(* Logix 5000 AddOnInstructionDefinition export DCO_WriteDriveParameter; software revision 20.01 *)

ADD_ON_INSTRUCTION DCO_WriteDriveParameter   (* revision 1.0 *)
// Write values to parameters in drive with data type INT and UINT
VAR_INPUT
   Instance_Number_Write : INT := 10518; {visible}
   Attribute_Number_Write : INT; {visible}
   Parameter_Value_Write : INT := 660; {visible}
   REQ_LEN : INT; {visible}
   Value_Out : INT; {visible}
END_VAR
VAR_IN_OUT
   MSG_Out : MESSAGE; {required}
END_VAR

ROUTINE Logic   (* ladder *)
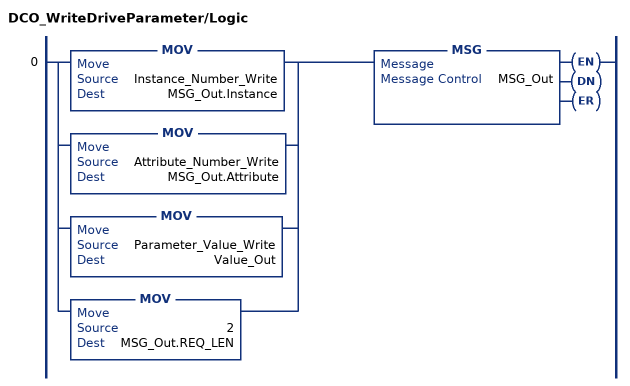
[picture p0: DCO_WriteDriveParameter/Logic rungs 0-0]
   0: [MOV(Instance_Number_Write,MSG_Out.Instance) ,[MOV(Attribute_Number_Write,MSG_Out.Attribute) ,[MOV(Parameter_Value_Write,Value_Out) ,MOV(2,MSG_Out.REQ_LEN) ] ] ]MSG(MSG_Out);
END_ROUTINE
END_ADD_ON_INSTRUCTION
